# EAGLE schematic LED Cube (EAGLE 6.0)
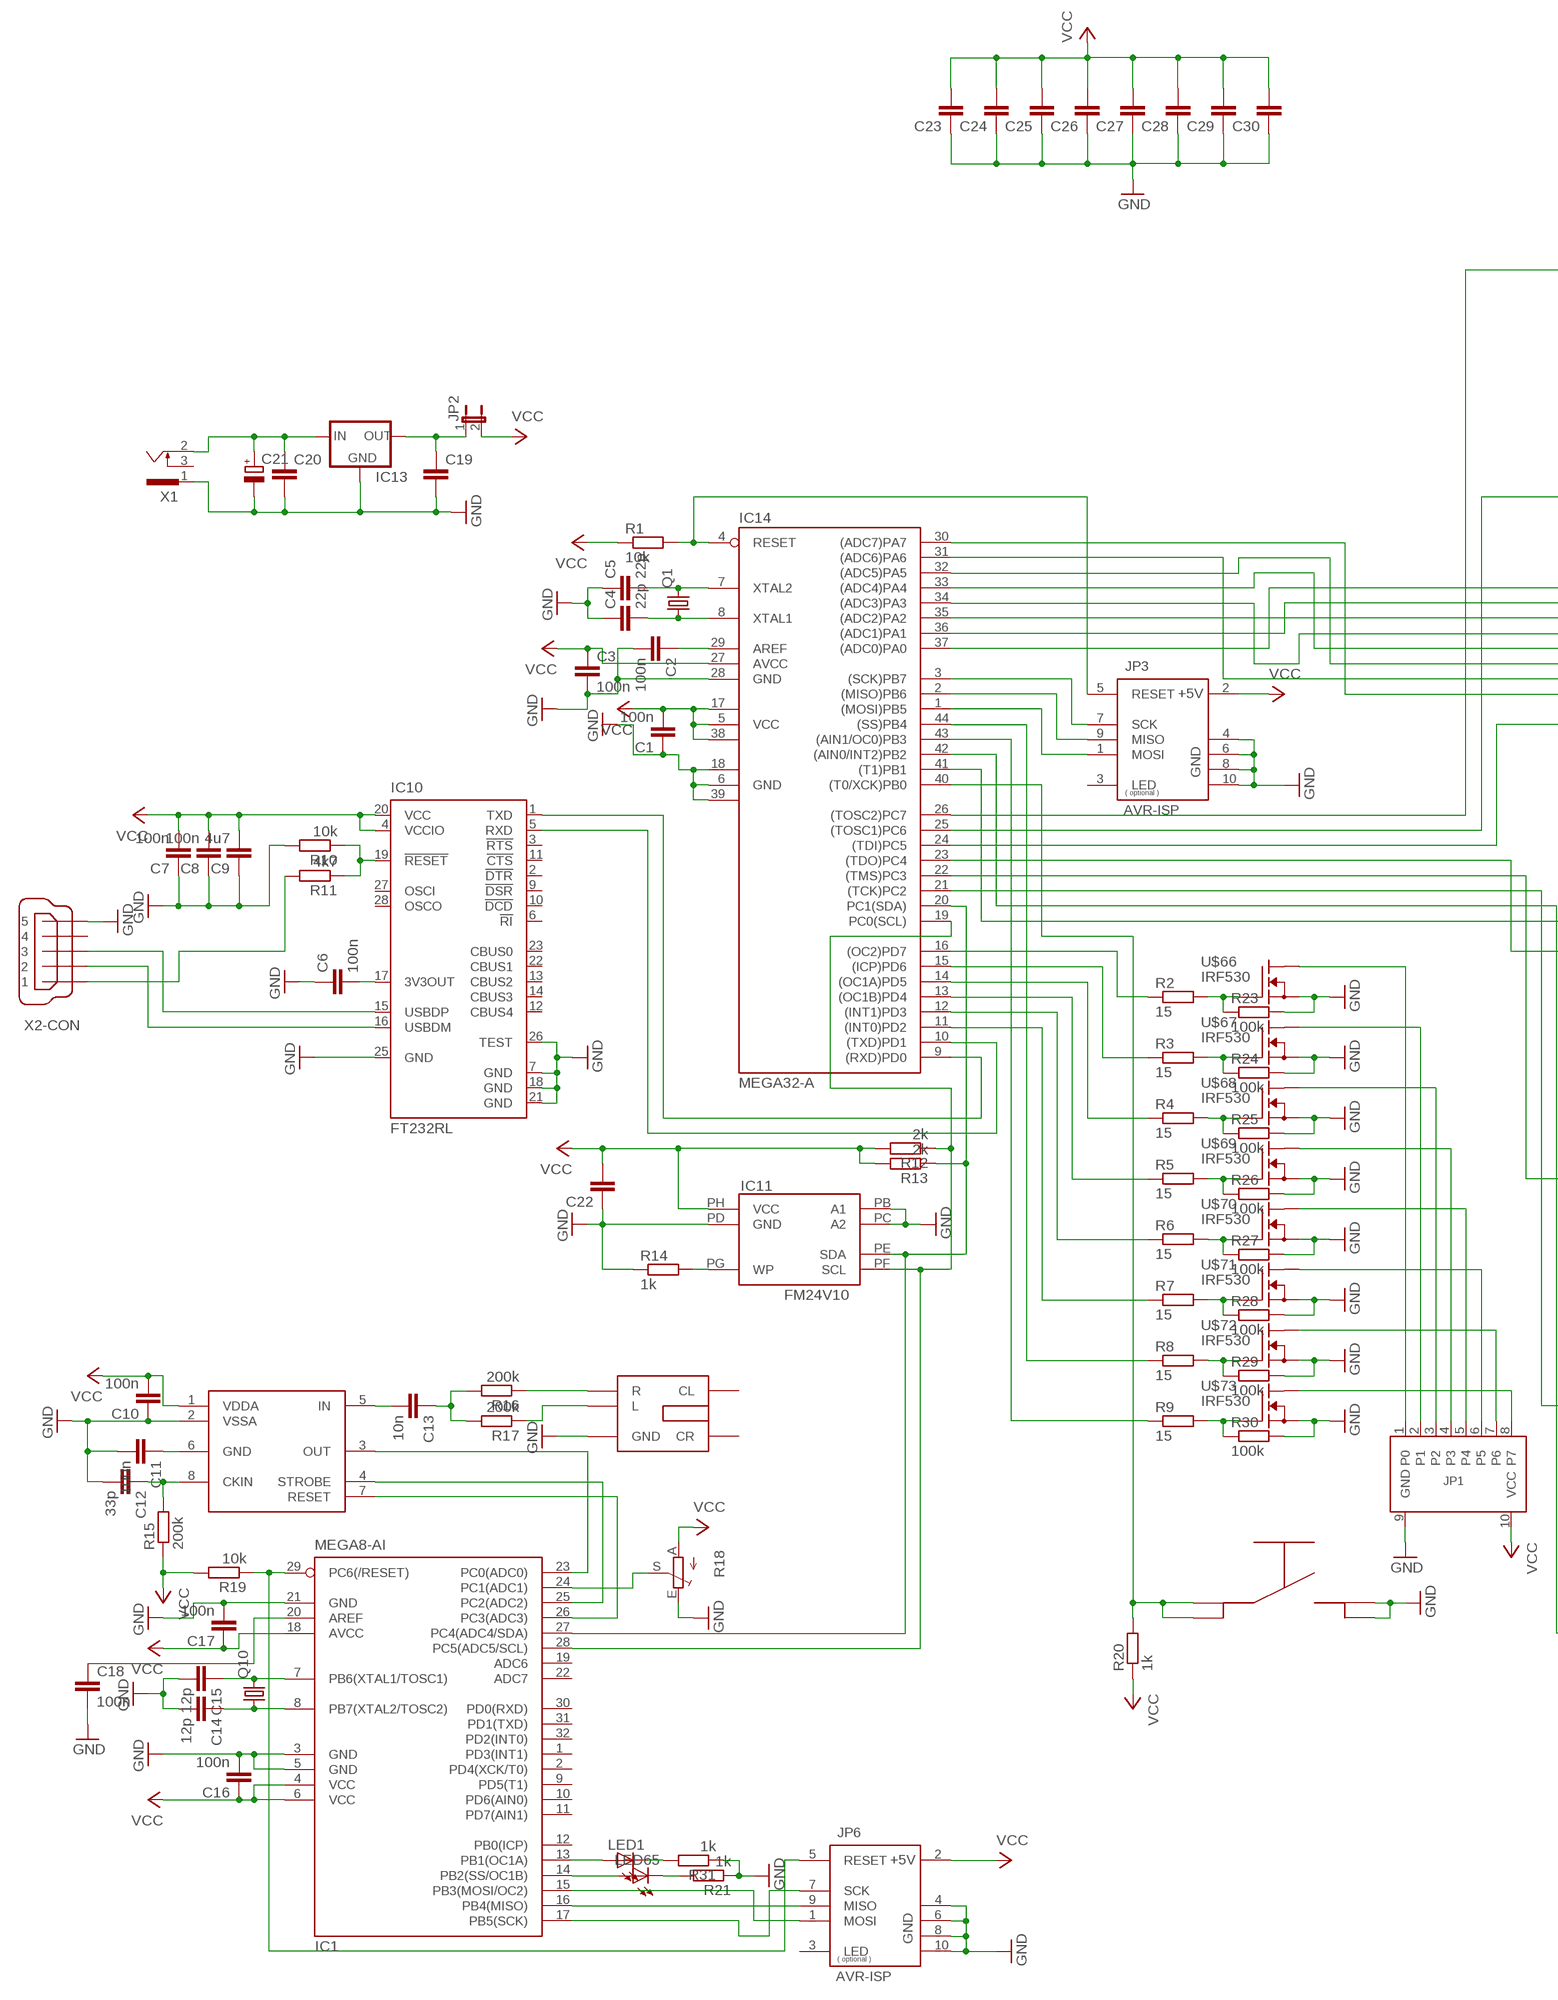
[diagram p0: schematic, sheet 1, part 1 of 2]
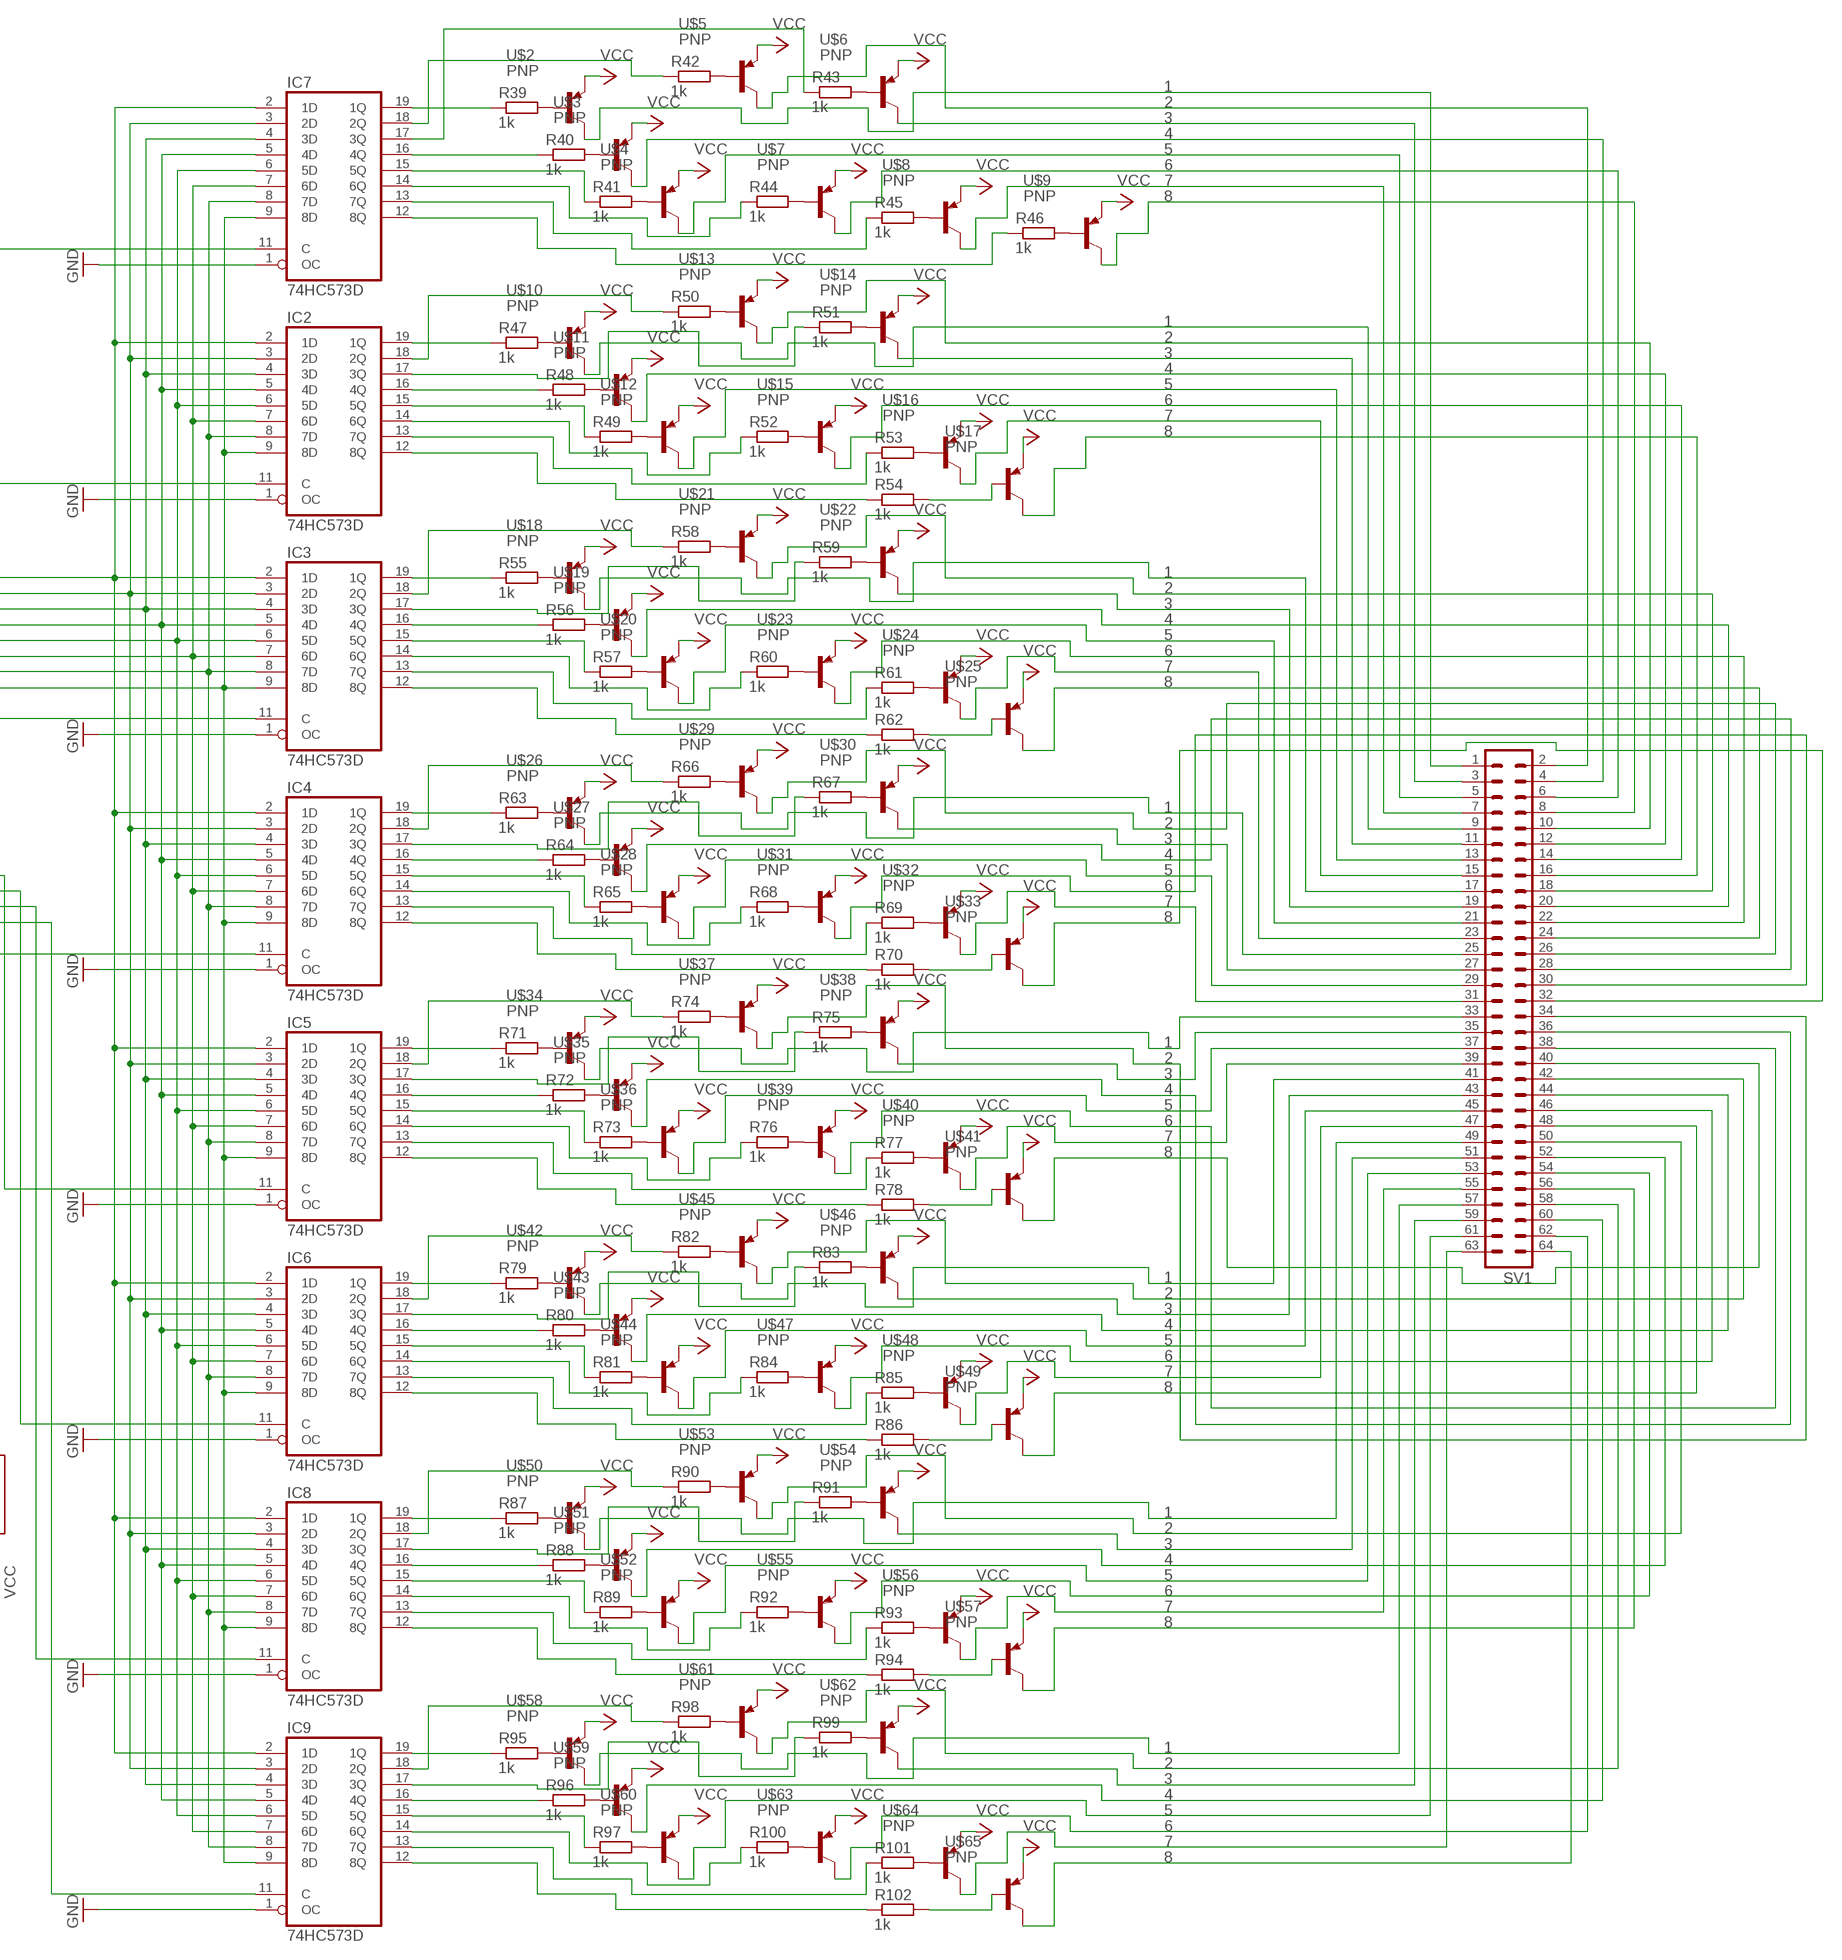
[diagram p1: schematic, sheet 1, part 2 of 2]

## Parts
C1  100n  C-EUC0603  [C0603]
C2  100n  C-EUC0603  [C0603]
C3  100n  C-EUC0603  [C0603]
C4  22p  C-EUC0603  [C0603]
C5  22p  C-EUC0603  [C0603]
C6  100n  C-EUC0603  [C0603]
C7  100n  C-EUC0603  [C0603]
C8  100n  C-EUC0603  [C0603]
C9  4u7  C-EUC0603  [C0603]
C10  100n  C-EUC0603  [C0603]
C11  100n  C-EUC0603  [C0603]
C12  33p  C-EUC0603  [C0603]
C13  10n  C-EUC0603  [C0603]
C14  12p  C-EUC0603  [C0603]
C15  12p  C-EUC0603  [C0603]
C16  100n  C-EUC0603  [C0603]
C17  100n  C-EUC0603  [C0603]
C18  100n  C-EUC0603  [C0603]
C19  C-EUC0603  [C0603]
C20  C-EUC0603  [C0603]
C21  CPOL-EUTAP5-80  [TAP5-80]
C22  C-EUC0603  [C0603]
C23  C-EUC0603  [C0603]
C24  C-EUC0603  [C0603]
C25  C-EUC0603  [C0603]
C26  C-EUC0603  [C0603]
C27  C-EUC0603  [C0603]
C28  C-EUC0603  [C0603]
C29  C-EUC0603  [C0603]
C30  C-EUC0603  [C0603]
IC1  MEGA8-AI  [TQFP32-08]
IC2  74HC573D  [SO20W]
IC3  74HC573D  [SO20W]
IC4  74HC573D  [SO20W]
IC5  74HC573D  [SO20W]
IC6  74HC573D  [SO20W]
IC7  74HC573D  [SO20W]
IC8  74HC573D  [SO20W]
IC9  74HC573D  [SO20W]
IC10  FT232RL  [SSOP28]
IC11  FM24V10  [SOIC8]
IC12  MSGEQ7  [DIP8]
IC13  78XXS  [78XXS]
IC14  MEGA32-A  [TQFP44]
JP1  PORT  [ML10]
JP2  JP1E  [JP1]
JP3  AVR-ISP  [ML10]
JP6  AVR-ISP  [ML10]
LED1  LEDCHIPLED_0603  [CHIPLED_0603]
LED65  LEDCHIPLED_0603  [CHIPLED_0603]
Q1  CRYSTALHC49S  [HC49/S]
Q10  CRYSTALHC49S  [HC49/S]
R1  10k  R-EU_R0603  [R0603]
R2  15  R-EU_R0603  [R0603]
R3  15  R-EU_R0603  [R0603]
R4  15  R-EU_R0603  [R0603]
R5  15  R-EU_R0603  [R0603]
R6  15  R-EU_R0603  [R0603]
R7  15  R-EU_R0603  [R0603]
R8  15  R-EU_R0603  [R0603]
R9  15  R-EU_R0603  [R0603]
R10  10k  R-EU_R0603  [R0603]
R11  4k7  R-EU_R0603  [R0603]
R12  2k  R-EU_R0603  [R0603]
R13  2k  R-EU_R0603  [R0603]
R14  1k  R-EU_R0603  [R0603]
R15  200k  R-EU_R0603  [R0603]
R16  200k  R-EU_R0603  [R0603]
R17  200k  R-EU_R0603  [R0603]
R18  TRIM_EU-PT10S  [PT-10S]
R19  10k  R-EU_R0603  [R0603]
R20  1k  R-EU_R0603  [R0603]
R21  1k  R-EU_R0603  [R0603]
R23  100k  R-EU_R0603  [R0603]
R24  100k  R-EU_R0603  [R0603]
R25  100k  R-EU_R0603  [R0603]
R26  100k  R-EU_R0603  [R0603]
R27  100k  R-EU_R0603  [R0603]
R28  100k  R-EU_R0603  [R0603]
R29  100k  R-EU_R0603  [R0603]
R30  100k  R-EU_R0603  [R0603]
R31  1k  R-EU_R0603  [R0603]
R39  1k  R-EU_R0603  [R0603]
R40  1k  R-EU_R0603  [R0603]
R41  1k  R-EU_R0603  [R0603]
R42  1k  R-EU_R0603  [R0603]
R43  1k  R-EU_R0603  [R0603]
R44  1k  R-EU_R0603  [R0603]
R45  1k  R-EU_R0603  [R0603]
R46  1k  R-EU_R0603  [R0603]
R47  1k  R-EU_R0603  [R0603]
R48  1k  R-EU_R0603  [R0603]
R49  1k  R-EU_R0603  [R0603]
R50  1k  R-EU_R0603  [R0603]
R51  1k  R-EU_R0603  [R0603]
R52  1k  R-EU_R0603  [R0603]
R53  1k  R-EU_R0603  [R0603]
R54  1k  R-EU_R0603  [R0603]
R55  1k  R-EU_R0603  [R0603]
R56  1k  R-EU_R0603  [R0603]
R57  1k  R-EU_R0603  [R0603]
R58  1k  R-EU_R0603  [R0603]
R59  1k  R-EU_R0603  [R0603]
R60  1k  R-EU_R0603  [R0603]
R61  1k  R-EU_R0603  [R0603]
R62  1k  R-EU_R0603  [R0603]
R63  1k  R-EU_R0603  [R0603]
R64  1k  R-EU_R0603  [R0603]
R65  1k  R-EU_R0603  [R0603]
R66  1k  R-EU_R0603  [R0603]
R67  1k  R-EU_R0603  [R0603]
R68  1k  R-EU_R0603  [R0603]
R69  1k  R-EU_R0603  [R0603]
R70  1k  R-EU_R0603  [R0603]
R71  1k  R-EU_R0603  [R0603]
R72  1k  R-EU_R0603  [R0603]
R73  1k  R-EU_R0603  [R0603]
R74  1k  R-EU_R0603  [R0603]
R75  1k  R-EU_R0603  [R0603]
R76  1k  R-EU_R0603  [R0603]
R77  1k  R-EU_R0603  [R0603]
R78  1k  R-EU_R0603  [R0603]
R79  1k  R-EU_R0603  [R0603]
R80  1k  R-EU_R0603  [R0603]
R81  1k  R-EU_R0603  [R0603]
R82  1k  R-EU_R0603  [R0603]
R83  1k  R-EU_R0603  [R0603]
R84  1k  R-EU_R0603  [R0603]
R85  1k  R-EU_R0603  [R0603]
R86  1k  R-EU_R0603  [R0603]
R87  1k  R-EU_R0603  [R0603]
R88  1k  R-EU_R0603  [R0603]
R89  1k  R-EU_R0603  [R0603]
R90  1k  R-EU_R0603  [R0603]
R91  1k  R-EU_R0603  [R0603]
R92  1k  R-EU_R0603  [R0603]
R93  1k  R-EU_R0603  [R0603]
R94  1k  R-EU_R0603  [R0603]
R95  1k  R-EU_R0603  [R0603]
R96  1k  R-EU_R0603  [R0603]
R97  1k  R-EU_R0603  [R0603]
R98  1k  R-EU_R0603  [R0603]
R99  1k  R-EU_R0603  [R0603]
R100  1k  R-EU_R0603  [R0603]
R101  1k  R-EU_R0603  [R0603]
R102  1k  R-EU_R0603  [R0603]
SV1  ML64  [ML64]
U$1  KLINKENBUCHSE  [KLINKEPRINT]
U$2  PNP  [SOT323]
U$3  PNP  [SOT323]
U$4  PNP  [SOT323]
U$5  PNP  [SOT323]
U$6  PNP  [SOT323]
U$7  PNP  [SOT323]
U$8  PNP  [SOT323]
U$9  PNP  [SOT323]
U$10  PNP  [SOT323]
U$11  PNP  [SOT323]
U$12  PNP  [SOT323]
U$13  PNP  [SOT323]
U$14  PNP  [SOT323]
U$15  PNP  [SOT323]
U$16  PNP  [SOT323]
U$17  PNP  [SOT323]
U$18  PNP  [SOT323]
U$19  PNP  [SOT323]
U$20  PNP  [SOT323]
U$21  PNP  [SOT323]
U$22  PNP  [SOT323]
U$23  PNP  [SOT323]
U$24  PNP  [SOT323]
U$25  PNP  [SOT323]
U$26  PNP  [SOT323]
U$27  PNP  [SOT323]
U$28  PNP  [SOT323]
U$29  PNP  [SOT323]
U$30  PNP  [SOT323]
U$31  PNP  [SOT323]
U$32  PNP  [SOT323]
U$33  PNP  [SOT323]
U$34  PNP  [SOT323]
U$35  PNP  [SOT323]
U$36  PNP  [SOT323]
U$37  PNP  [SOT323]
U$38  PNP  [SOT323]
U$39  PNP  [SOT323]
U$40  PNP  [SOT323]
U$41  PNP  [SOT323]
U$42  PNP  [SOT323]
U$43  PNP  [SOT323]
U$44  PNP  [SOT323]
U$45  PNP  [SOT323]
U$46  PNP  [SOT323]
U$47  PNP  [SOT323]
U$48  PNP  [SOT323]
U$49  PNP  [SOT323]
U$50  PNP  [SOT323]
U$51  PNP  [SOT323]
U$52  PNP  [SOT323]
U$53  PNP  [SOT323]
U$54  PNP  [SOT323]
U$55  PNP  [SOT323]
U$56  PNP  [SOT323]
U$57  PNP  [SOT323]
U$58  PNP  [SOT323]
U$59  PNP  [SOT323]
U$60  PNP  [SOT323]
U$61  PNP  [SOT323]
U$62  PNP  [SOT323]
U$63  PNP  [SOT323]
U$64  PNP  [SOT323]
U$65  PNP  [SOT323]
U$66  IRF530  [TO220-3V]
U$67  IRF530  [TO220-3V]
U$68  IRF530  [TO220-3V]
U$69  IRF530  [TO220-3V]
U$70  IRF530  [TO220-3V]
U$71  IRF530  [TO220-3V]
U$72  IRF530  [TO220-3V]
U$73  IRF530  [TO220-3V]
U$74  TASTER  [SMDTASTER]
X1  733980-62  [733980-62]
X2  USB-B-MINI-SMD  [USB-B-MINI-SMD]

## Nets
GND: C1.1 C2.2 C3.2 C4.1 C5.1 C6.1 C7.1 C8.1 C9.1 C10.1 C11.2 C12.2 C14.2 C15.2 C16.2 C17.2 C18.2 C19.2 C20.2 C21.- C22.1 C23.1 C24.1 C25.1 C26.1 C27.1 C28.1 C29.1 C30.1 IC1.3(GND) IC1.5(GND) IC1.21(GND) IC2.1(OC) IC3.1(OC) IC4.1(OC) IC5.1(OC) IC6.1(OC) IC7.1(OC) IC8.1(OC) IC9.1(OC) IC10.7(GND) IC10.18(GND) IC10.21(GND) IC10.25(GND) IC10.26(TEST) IC11.PB(A1) IC11.PC(A2) IC11.PD(GND) IC12.2(VSSA) IC13.GND IC14.6(GND) IC14.18(GND1) IC14.28(GND) IC14.39(GND2) JP1.9(GND) JP3.4(GND) JP3.6(GND) JP3.8(GND) JP3.10(GND) JP6.4(GND) JP6.6(GND) JP6.8(GND) JP6.10(GND) R10.2 R14.1 R18.E R21.1 R23.2 R24.2 R25.2 R26.2 R27.2 R28.2 R29.2 R30.2 R31.1 U$1.GND U$66.3(S) U$67.3(S) U$68.3(S) U$69.3(S) U$70.3(S) U$71.3(S) U$72.3(S) U$73.3(S) U$74.B U$74.B2 X1.1 X2.5
N$1: SV1.4 U$3.P$3(C)
N$2: IC14.4(RESET) JP3.5(RESET) R1.2
N$3: C2.1 IC14.29(AREF)
N$4: IC2.2(1D) IC3.2(1D) IC4.2(1D) IC5.2(1D) IC6.2(1D) IC7.2(1D) IC8.2(1D) IC9.2(1D) IC14.37((ADC0)PA0)
N$5: IC2.3(2D) IC3.3(2D) IC4.3(2D) IC5.3(2D) IC6.3(2D) IC7.3(2D) IC8.3(2D) IC9.3(2D) IC14.36((ADC1)PA1)
N$6: IC2.4(3D) IC3.4(3D) IC4.4(3D) IC5.4(3D) IC6.4(3D) IC7.4(3D) IC8.4(3D) IC9.4(3D) IC14.35((ADC2)PA2)
N$7: C5.2 IC14.7(XTAL2) Q1.2
N$8: C4.2 IC14.8(XTAL1) Q1.1
N$9: IC2.5(4D) IC3.5(4D) IC4.5(4D) IC5.5(4D) IC6.5(4D) IC7.5(4D) IC8.5(4D) IC9.5(4D) IC14.34((ADC3)PA3)
N$10: IC2.6(5D) IC3.6(5D) IC4.6(5D) IC5.6(5D) IC6.6(5D) IC7.6(5D) IC8.6(5D) IC9.6(5D) IC14.33((ADC4)PA4)
N$11: IC2.7(6D) IC3.7(6D) IC4.7(6D) IC5.7(6D) IC6.7(6D) IC7.7(6D) IC8.7(6D) IC9.7(6D) IC14.32((ADC5)PA5)
N$12: IC2.8(7D) IC3.8(7D) IC4.8(7D) IC5.8(7D) IC6.8(7D) IC7.8(7D) IC8.8(7D) IC9.8(7D) IC14.31((ADC6)PA6)
N$13: IC2.9(8D) IC3.9(8D) IC4.9(8D) IC5.9(8D) IC6.9(8D) IC7.9(8D) IC8.9(8D) IC9.9(8D) IC14.30((ADC7)PA7)
N$14: IC9.11(C) IC14.41((T1)PB1)
N$15: IC8.11(C) IC14.42((AIN0/INT2)PB2)
N$16: IC6.11(C) IC14.21((TCK)PC2)
N$17: IC5.11(C) IC14.22((TMS)PC3)
N$18: IC4.11(C) IC14.23((TDO)PC4)
N$19: IC3.11(C) IC14.24((TDI)PC5)
N$20: IC2.11(C) IC14.25((TOSC1)PC6)
N$21: IC7.11(C) IC14.26((TOSC2)PC7)
N$22: R2.2 R23.1 U$66.1(G)
N$23: IC14.16((OC2)PD7) R2.1
N$24: IC14.15((ICP)PD6) R3.1
N$25: IC14.14((OC1A)PD5) R4.1
N$26: IC14.13((OC1B)PD4) R5.1
N$27: IC14.12((INT1)PD3) R6.1
N$28: IC14.11((INT0)PD2) R7.1
N$29: IC14.44((SS)PB4) R8.1
N$30: IC14.43((AIN1/OC0)PB3) R9.1
N$31: R3.2 R24.1 U$67.1(G)
N$32: R4.2 R25.1 U$68.1(G)
N$33: R5.2 R26.1 U$69.1(G)
N$34: R6.2 R27.1 U$70.1(G)
N$35: R7.2 R28.1 U$71.1(G)
N$36: R8.2 R29.1 U$72.1(G)
N$37: R9.2 R30.1 U$73.1(G)
N$38: JP1.1(P0) U$66.2(D)
N$39: JP1.2(P1) U$67.2(D)
N$42: JP1.5(P4) U$70.2(D)
N$43: JP1.6(P5) U$71.2(D)
N$44: JP1.7(P6) U$72.2(D)
N$45: JP1.8(P7) U$73.2(D)
N$46: R11.2 X2.1
N$47: IC14.3((SCK)PB7) JP3.7(SCK)
N$48: IC14.2((MISO)PB6) JP3.9(MISO)
N$49: IC14.1((MOSI)PB5) JP3.1(MOSI)
N$50: IC10.5(RXD) IC14.10((TXD)PD1)
N$51: IC10.1(TXD) IC14.9((RXD)PD0)
N$52: IC10.19(!RESET) R10.1 R11.1
N$53: IC1.27(PC4(ADC4/SDA)) IC11.PE(SDA) IC14.20(PC1(SDA)) R13.1
N$54: IC10.15(USBDP) X2.3
N$55: C6.2 IC10.17(3V3OUT)
N$56: IC10.16(USBDM) X2.2
N$57: IC1.28(PC5(ADC5/SCL)) IC11.PF(SCL) IC14.19(PC0(SCL)) R12.1
N$58: IC11.PG(WP) R14.2
N$59: C12.1 IC12.8(CKIN) R15.2
N$60: C11.1 IC12.6(GND)
N$61: C13.2 IC12.5(IN)
N$62: C13.1 R16.2 R17.2
N$63: R16.1 U$1.RIGHT(R)
N$64: R17.1 U$1.LEFT(L)
N$65: IC1.23(PC0(ADC0)) IC12.3(OUT)
N$66: IC1.29(PC6(/RESET)) JP6.5(RESET) R19.1
N$67: IC1.25(PC2(ADC2)) IC12.4(STROBE)
N$68: IC1.26(PC3(ADC3)) IC12.7(RESET)
N$69: IC14.40((T0/XCK)PB0) R20.2 U$74.A U$74.A2
N$70: C14.1 IC1.8(PB7(XTAL2/TOSC2)) Q10.1
N$71: C15.1 IC1.7(PB6(XTAL1/TOSC1)) Q10.2
N$74: C20.1 C21.+ IC13.IN X1.2
N$75: IC1.14(PB2(SS/OC1B)) LED65.A
N$76: LED65.C R21.2
N$77: IC1.24(PC1(ADC1)) R18.S
N$78: C18.1 IC1.20(AREF)
N$79: IC1.16(PB4(MISO)) JP6.9(MISO)
N$80: IC1.15(PB3(MOSI/OC2)) JP6.1(MOSI)
N$81: IC1.17(PB5(SCK)) JP6.7(SCK)
N$82: LED1.C R31.2
N$83: IC1.13(PB1(OC1A)) LED1.A
N$84: C19.1 IC13.OUT JP2.1
N$98: SV1.2 U$5.P$3(C)
N$99: SV1.3 U$6.P$3(C)
N$100: SV1.5 U$4.P$3(C)
N$101: R44.2 U$7.P$1(B)
N$102: SV1.6 U$7.P$3(C)
N$103: R42.2 U$5.P$1(B)
N$104: SV1.8 U$9.P$3(C)
N$105: SV1.16 U$17.P$3(C)
N$106: R63.2 U$26.P$1(B)
N$107: R64.2 U$27.P$1(B)
N$108: R65.2 U$28.P$1(B)
N$109: SV1.12 U$11.P$3(C)
N$110: SV1.10 U$13.P$3(C)
N$111: SV1.9 U$10.P$3(C)
N$112: R54.2 U$17.P$1(B)
N$113: IC4.19(1Q) R63.1
N$114: IC4.16(4Q) R64.1
N$115: R66.2 U$29.P$1(B)
N$116: IC4.18(2Q) R66.1
N$117: R67.2 U$30.P$1(B)
N$118: IC4.17(3Q) R67.1
N$119: IC4.15(5Q) R65.1
N$120: R68.2 U$31.P$1(B)
N$121: R71.2 U$34.P$1(B)
N$122: R72.2 U$35.P$1(B)
N$123: R73.2 U$36.P$1(B)
N$124: IC5.19(1Q) R71.1
N$125: IC5.16(4Q) R72.1
N$126: R74.2 U$37.P$1(B)
N$127: IC5.18(2Q) R74.1
N$128: R75.2 U$38.P$1(B)
N$129: IC7.19(1Q) R39.1
N$130: SV1.63 U$64.P$3(C)
N$131: SV1.61 U$60.P$3(C)
N$132: IC7.16(4Q) R40.1
N$133: IC2.19(1Q) R47.1
N$134: SV1.62 U$63.P$3(C)
N$135: IC2.16(4Q) R48.1
N$136: SV1.58 U$61.P$3(C)
N$137: R95.2 U$58.P$1(B)
N$138: SV1.55 U$56.P$3(C)
N$139: R96.2 U$59.P$1(B)
N$140: R97.2 U$60.P$1(B)
N$141: IC9.19(1Q) R95.1
N$142: SV1.54 U$55.P$3(C)
N$143: IC9.16(4Q) R96.1
N$144: SV1.50 U$53.P$3(C)
N$145: R87.2 U$50.P$1(B)
N$146: R88.2 U$51.P$1(B)
N$147: R89.2 U$52.P$1(B)
N$148: IC8.16(4Q) R88.1
N$149: IC8.19(1Q) R87.1
N$150: R90.2 U$53.P$1(B)
N$151: IC8.18(2Q) R90.1
N$152: R91.2 U$54.P$1(B)
N$153: R79.2 U$42.P$1(B)
N$154: R80.2 U$43.P$1(B)
N$155: R81.2 U$44.P$1(B)
N$156: IC6.19(1Q) R79.1
N$157: IC6.16(4Q) R80.1
N$158: R82.2 U$45.P$1(B)
N$159: IC6.18(2Q) R82.1
N$160: R83.2 U$46.P$1(B)
N$161: R40.2 U$3.P$1(B)
N$162: R39.2 U$2.P$1(B)
N$163: IC7.15(5Q) R41.1
N$164: SV1.1 U$2.P$3(C)
N$165: R41.2 U$4.P$1(B)
N$166: SV1.7 U$8.P$3(C)
N$167: IC3.19(1Q) R55.1
N$168: IC3.16(4Q) R56.1
N$169: R47.2 U$10.P$1(B)
N$170: IC7.14(6Q) R44.1
N$171: R45.2 U$8.P$1(B)
N$172: IC7.18(2Q) R42.1
N$173: R43.2 U$6.P$1(B)
N$174: R48.2 U$11.P$1(B)
N$175: IC7.17(3Q) R43.1
N$176: IC7.13(7Q) R45.1
N$177: R46.2 U$9.P$1(B)
N$178: R49.2 U$12.P$1(B)
N$179: IC7.12(8Q) R46.1
N$180: SV1.17 U$18.P$3(C)
N$181: SV1.25 U$26.P$3(C)
N$182: IC4.14(6Q) R68.1
N$183: SV1.13 U$12.P$3(C)
N$184: R50.2 U$13.P$1(B)
N$185: IC2.18(2Q) R50.1
N$186: R51.2 U$14.P$1(B)
N$187: IC2.17(3Q) R51.1
N$188: SV1.11 U$14.P$3(C)
N$189: IC2.15(5Q) R49.1
N$190: R69.2 U$32.P$1(B)
N$191: IC4.13(7Q) R69.1
N$192: R52.2 U$15.P$1(B)
N$193: IC2.14(6Q) R52.1
N$194: SV1.14 U$15.P$3(C)
N$195: R53.2 U$16.P$1(B)
N$196: IC2.13(7Q) R53.1
N$197: SV1.15 U$16.P$3(C)
N$198: IC4.12(8Q) R70.1
N$199: SV1.32 U$33.P$3(C)
N$200: IC2.12(8Q) R54.1
N$201: R55.2 U$18.P$1(B)
N$202: R56.2 U$19.P$1(B)
N$203: R57.2 U$20.P$1(B)
N$204: SV1.33 U$34.P$3(C)
N$205: SV1.41 U$42.P$3(C)
N$206: R58.2 U$21.P$1(B)
N$207: IC3.18(2Q) R58.1
N$208: R59.2 U$22.P$1(B)
N$209: IC3.17(3Q) R59.1
N$210: IC3.15(5Q) R57.1
N$211: R60.2 U$23.P$1(B)
N$212: IC3.14(6Q) R60.1
N$213: R61.2 U$24.P$1(B)
N$214: IC3.13(7Q) R61.1
N$215: IC3.12(8Q) R62.1
N$216: SV1.24 U$25.P$3(C)
N$217: SV1.23 U$24.P$3(C)
N$218: SV1.22 U$23.P$3(C)
N$219: SV1.21 U$20.P$3(C)
N$220: SV1.20 U$19.P$3(C)
N$221: SV1.18 U$21.P$3(C)
N$222: SV1.49 U$50.P$3(C)
N$223: R62.2 U$25.P$1(B)
N$224: SV1.19 U$22.P$3(C)
N$225: SV1.31 U$32.P$3(C)
N$226: SV1.30 U$31.P$3(C)
N$227: SV1.29 U$28.P$3(C)
N$228: SV1.28 U$27.P$3(C)
N$229: SV1.26 U$29.P$3(C)
N$230: SV1.57 U$58.P$3(C)
N$231: R70.2 U$33.P$1(B)
N$232: SV1.27 U$30.P$3(C)
N$233: IC5.17(3Q) R75.1
N$234: IC5.15(5Q) R73.1
N$235: R76.2 U$39.P$1(B)
N$236: IC5.14(6Q) R76.1
N$237: R77.2 U$40.P$1(B)
N$238: IC5.13(7Q) R77.1
N$239: IC5.12(8Q) R78.1
N$240: SV1.40 U$41.P$3(C)
N$241: SV1.39 U$40.P$3(C)
N$242: SV1.38 U$39.P$3(C)
N$243: SV1.37 U$36.P$3(C)
N$244: SV1.36 U$35.P$3(C)
N$245: SV1.34 U$37.P$3(C)
N$247: R78.2 U$41.P$1(B)
N$248: SV1.35 U$38.P$3(C)
N$249: IC6.17(3Q) R83.1
N$250: IC6.15(5Q) R81.1
N$251: R84.2 U$47.P$1(B)
N$252: IC6.14(6Q) R84.1
N$253: R85.2 U$48.P$1(B)
N$254: IC6.13(7Q) R85.1
N$255: IC6.12(8Q) R86.1
N$256: SV1.48 U$49.P$3(C)
N$257: SV1.47 U$48.P$3(C)
N$258: SV1.46 U$47.P$3(C)
N$259: SV1.45 U$44.P$3(C)
N$260: SV1.44 U$43.P$3(C)
N$261: SV1.42 U$45.P$3(C)
N$263: R86.2 U$49.P$1(B)
N$264: SV1.43 U$46.P$3(C)
N$265: IC8.17(3Q) R91.1
N$266: IC8.15(5Q) R89.1
N$267: R92.2 U$55.P$1(B)
N$268: IC8.14(6Q) R92.1
N$269: R93.2 U$56.P$1(B)
N$270: IC8.13(7Q) R93.1
N$271: IC8.12(8Q) R94.1
N$272: SV1.56 U$57.P$3(C)
N$273: R98.2 U$61.P$1(B)
N$274: IC9.18(2Q) R98.1
N$275: SV1.53 U$52.P$3(C)
N$276: SV1.52 U$51.P$3(C)
N$277: R99.2 U$62.P$1(B)
N$278: JP1.3(P2) U$68.2(D)
N$279: R94.2 U$57.P$1(B)
N$280: SV1.51 U$54.P$3(C)
N$281: IC9.17(3Q) R99.1
N$282: IC9.15(5Q) R97.1
N$283: R100.2 U$63.P$1(B)
N$284: IC9.14(6Q) R100.1
N$285: R101.2 U$64.P$1(B)
N$286: IC9.13(7Q) R101.1
N$287: IC9.12(8Q) R102.1
N$288: SV1.64 U$65.P$3(C)
N$289: JP1.4(P3) U$69.2(D)
N$292: SV1.60 U$59.P$3(C)
N$295: R102.2 U$65.P$1(B)
N$296: SV1.59 U$62.P$3(C)
VCC: C1.2 C3.1 C7.2 C8.2 C9.2 C10.2 C16.1 C17.1 C22.2 C23.2 C24.2 C25.2 C26.2 C27.2 C28.2 C29.2 C30.2 IC1.4(VCC) IC1.6(VCC) IC1.18(AVCC) IC10.4(VCCIO) IC10.20(VCC) IC11.PH(VCC) IC12.1(VDDA) IC14.5(VCC) IC14.17(VCC1) IC14.27(AVCC) IC14.38(VCC2) JP1.10(VCC) JP2.2 JP3.2(+5V) JP6.2(+5V) R1.1 R12.2 R13.2 R15.1 R18.A R19.2 R20.1 U$2.P$2(E) U$3.P$2(E) U$4.P$2(E) U$5.P$2(E) U$6.P$2(E) U$7.P$2(E) U$8.P$2(E) U$9.P$2(E) U$10.P$2(E) U$11.P$2(E) U$12.P$2(E) U$13.P$2(E) U$14.P$2(E) U$15.P$2(E) U$16.P$2(E) U$17.P$2(E) U$18.P$2(E) U$19.P$2(E) U$20.P$2(E) U$21.P$2(E) U$22.P$2(E) U$23.P$2(E) U$24.P$2(E) U$25.P$2(E) U$26.P$2(E) U$27.P$2(E) U$28.P$2(E) U$29.P$2(E) U$30.P$2(E) U$31.P$2(E) U$32.P$2(E) U$33.P$2(E) U$34.P$2(E) U$35.P$2(E) U$36.P$2(E) U$37.P$2(E) U$38.P$2(E) U$39.P$2(E) U$40.P$2(E) U$41.P$2(E) U$42.P$2(E) U$43.P$2(E) U$44.P$2(E) U$45.P$2(E) U$46.P$2(E) U$47.P$2(E) U$48.P$2(E) U$49.P$2(E) U$50.P$2(E) U$51.P$2(E) U$52.P$2(E) U$53.P$2(E) U$54.P$2(E) U$55.P$2(E) U$56.P$2(E) U$57.P$2(E) U$58.P$2(E) U$59.P$2(E) U$60.P$2(E) U$61.P$2(E) U$62.P$2(E) U$63.P$2(E) U$64.P$2(E) U$65.P$2(E)
Unconnected: IC1.1(PD3(INT1)) IC1.2(PD4(XCK/T0)) IC1.9(PD5(T1)) IC1.10(PD6(AIN0)) IC1.11(PD7(AIN1)) IC1.12(PB0(ICP)) IC1.19(ADC6) IC1.22(ADC7) IC1.30(PD0(RXD)) IC1.31(PD1(TXD)) IC1.32(PD2(INT0)) IC10.2(!DTR) IC10.3(!RTS) IC10.6(!RI) IC10.9(!DSR) IC10.10(!DCD) IC10.11(!CTS) IC10.12(CBUS4) IC10.13(CBUS2) IC10.14(CBUS3) IC10.22(CBUS1) IC10.23(CBUS0) IC10.27(OSCI) IC10.28(OSCO) JP3.3(LED) JP6.3(LED) U$1.CONLEFT(CL) U$1.CONRIGHT(CR) X1.3 X2.4 X2.M1(-SHIELD:S1) X2.M2(-SHIELD:S2) X2.M3(-SHIELD:S3) X2.M4(-SHIELD:S4)

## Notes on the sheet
- 1
- 2
- 3
- 4
- 5
- 6
- 7
- 8
- 1
- 2
- 3
- 4
- 5
- 6
- 7
- 8
- 1
- 2
- 3
- 4
- 5
- 6
- 7
- 8
- 1
- 2
- 3
- 4
- 5
- 6
- 7
- 8
- 1
- 2
- 3
- 4
- 5
- 6
- 7
- 8
- 1
- 2
- 3
- 4
- 5
- 6
- 7
- 8
- 1
- 2
- 3
- 4
- 5
- 6
- 7
- 8
- 1
- 2
- 3
- 4
- 5
- 6
- 7
- 8

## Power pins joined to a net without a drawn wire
GND: IC2.10(GND) IC3.10(GND) IC4.10(GND) IC5.10(GND) IC6.10(GND) IC7.10(GND) IC8.10(GND) IC9.10(GND)
VCC: IC2.20(VCC) IC3.20(VCC) IC4.20(VCC) IC5.20(VCC) IC6.20(VCC) IC7.20(VCC) IC8.20(VCC) IC9.20(VCC)

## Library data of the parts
C1-C20 C22-C30 = resistor:C-EU: CAPACITOR, European symbol
C21 = resistor:CPOL-EU: POLARIZED CAPACITOR, European symbol
IC1 = atmel:MEGA8: MICROCONTROLLER 8 Kbytes FLASH, 1 kbytes SRAM, 512 bytes EEPROM, USART, 6-channel 10 bit ADC, 2-channel 8 bit ADC Pin compatible with Atmega48, ATMega88, ATMega168 Source: avr.lbr; MPN: ATMEGA8-16AU; OC_FARNELL: 9171371; OC_NEWARK: 73M8863
IC2-IC9 = 74xx-eu:74*573: 8-bit D latch BUS DRIVER
IC10 = ftdichip:FT232R: Source: http://www.ftdichip.com/Documents/DataSheets/DS_FT232R_v104.pdf; MPN: FT232RL; OC_FARNELL: 1146032; OC_NEWARK: 91K9918
IC11 = 0-xythobuz:FM24V10
IC12 = 0-xythobuz:MSGEQ7
IC13 = v-reg:78XXS: VOLTAGE REGULATOR
IC14 = atmel:MEGA32: MICROCONTROLLER 32 Kbytes FLASH 2 Kbytes SRAM 1 Kbytes EEPROM USART 8-channel 10 bit ADC Source: www.atmel.com .. doc2503.pdf; MPN: ATMEGA32-16AU; OC_FARNELL: 9171274; OC_NEWARK: 69K6677
JP1 = 0-roboternetz-definitionen:PORT: Datenportstecker Kompatibel zu den Steckern des STK500
JP2 = jumper:JP1E: JUMPER
JP3 JP6 = 0-roboternetz-definitionen:AVR-ISP: ISP ( In System Programming ) Stecker für AVRs Über diesen Anschluß kann ein AVR mit einem Standard ISP-Kabel direkt an einen Parallelport des PC´s angeschlossen und programmiert werden. Die Belegung des ISP-Anschlusses ist zu dem weit verbreitetet STK200 Programmier Dongle kompatibel. Ein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
LED1 LED65 = led:LED: LED
Q1 Q10 = crystal:CRYSTAL: CRYSTAL; OC_FARNELL: 1667008; OC_NEWARK: unknown
R1-R17 R19-R21 R23-R31 R39-R102 = resistor:R-EU_: RESISTOR, European symbol
R18 = pot:TRIM_EU-: POTENTIOMETER
SV1 = con-ml:ML64: HARTING; OC_FARNELL: unknown; OC_NEWARK: unknown
U$1 = 0-xythobuz:KLINKENBUCHSE: 3.5mm Klinkenbuchse, print. CL and CR are connected to left and right respectively, when no 3,5mm Klinkenstecker is inserted. If a stecker is plugged in, they have no connection.
U$2-U$65 = 0-xythobuz:PNP
U$66-U$73 = 0-xythobuz:IRF530
U$74 = 0-xythobuz:TASTER
X1 = con-conrad:73398?: FEMALE PRINT CONNECTOR Niedervolt-Steckverbinder Distributor Conrad
X2 = 1_USER:USB-B-MINI-SMD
